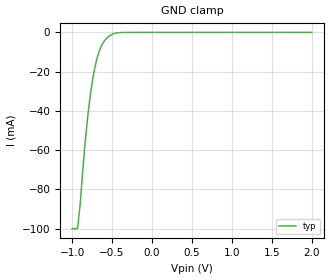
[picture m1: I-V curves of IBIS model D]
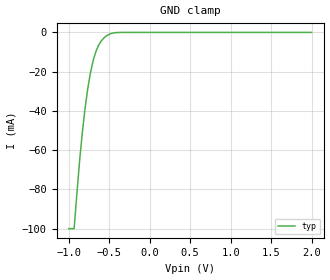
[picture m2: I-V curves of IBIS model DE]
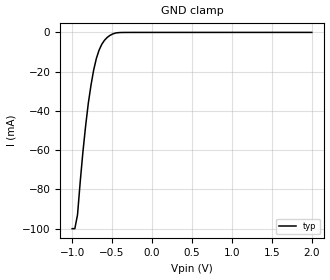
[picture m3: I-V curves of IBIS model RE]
| Texas Instruments Incorporated
| Dominant Mode Multipoint Transceiver
| Marketing part#   Voltage Range   Package-type   #pins/pkg drawing
| DS36277   4.75V - 5.25V   SOIC   8-pin D
[IBIS Ver]   4.1
[File name]   ds36277.ibs
[File Rev]   1.0
[Date]   10/01/2014
[Source]   Model built from bench measurements at:
   Texas Instruments Incorporated.
   Analog-eLab, HPA
   12500 TI Blvd
   Dallas, TX -75243
   For Support e-mail: elab_ibis@list.ti.com
[Notes]   Revision History
   Rev 1.0: 10/01/2014
   - ccomp values are based on measurement to GND.
   - R 3-state output Pullup is non-monotonic and as measured.
[Disclaimer]  This model is designed as an aid for customers of Texas Instruments
 TI and its licensors and suppliers make no warranties, either expressed
 or implied, with respect to this  model, including the warranties of
 merchantability or fitness for a particular purpose.
 The model is provided solely on an "as is" basis. The entire risk as to
 its quality and performance is with the customer.
[Copyright] (C)Copyright 2014 Texas Instruments Incorporated.
   All rights reserved.
[Component]   DS36277D
[Manufacturer]  Texas Instruments Incorporated
[Package]   |8-pin SOIC D package
|   typ   min   max
R_pkg   0   0   0
L_pkg   0   0   0
C_pkg   0   0   0
[Pin]   signal_name   model_name   R_pin   L_pin   C_pin
1   R   R
2   RE   RE
3   DE   DE
4   D   D
5   GND   GND
6   A   DO
7   B   DO
8   VCC1   POWER
[Diff pin]  inv_pin  vdiff  tdelay_typ  tdelay_min  tdelay_max
 6   7   0.0   0.0s   0.0s   0.0s
| Models and submodels in the file (5): D (Input), DE (Input), RE (Input), R (3-state), DO (I/O)
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|   Model D
[Model]   D
Model_type   Input
Vinl = .8
Vinh = 2
|   typ   min   max
|   (nom PVT)   (fast PVT)   (slow PVT)
C_comp   11.252pF   NA   NA
[Voltage Range]   5   NA   NA
[Temperature Range]   27   NA   NA
[Power Clamp Reference]   5   NA   NA
[GND Clamp Reference]   0   0   0
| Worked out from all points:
|   GND clamp passes 1 mA (typ) near -0.50 V on its own axis
[GND Clamp]
|   Voltage   I(typ)   I(min)  I(max)
-1V       -100mA     NA         NA
-932.6mV  -100mA     NA         NA
-898.9mV  -87.56mA   NA         NA
-865.2mV  -69.25mA   NA         NA
-831.5mV  -53.38mA   NA         NA
-797.8mV  -40.13mA   NA         NA
-764mV    -29.44mA   NA         NA
-730.3mV  -20.87mA   NA         NA
-662.9mV  -9.703mA   NA         NA
-561.8mV  -2.723mA   NA         NA
-359.6mV  -36.74uA   NA         NA
2V        0A         NA         NA
|   Model DE
[Model]   DE
Model_type   Input
Vinl = .8
Vinh = 2
|   typ   min   max
|   (nom PVT)   (fast PVT)   (slow PVT)
C_comp   11.252pF   NA   NA
[Voltage Range]   5   NA   NA
[Temperature Range]   27   NA   NA
[Power Clamp Reference]   5   NA   NA
[GND Clamp Reference]   0   0   0
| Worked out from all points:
|   GND clamp passes 1 mA (typ) near -0.50 V on its own axis
[GND Clamp]
|   Voltage   I(typ)   I(min)  I(max)
-1V       -100mA     NA         NA
-932.6mV  -100mA     NA         NA
-865.2mV  -65.53mA   NA         NA
-831.5mV  -51.06mA   NA         NA
-797.8mV  -38.77mA   NA         NA
-764mV    -28.58mA   NA         NA
-730.3mV  -20.45mA   NA         NA
-662.9mV  -9.664mA   NA         NA
-629.2mV  -6.458mA   NA         NA
-561.8mV  -2.706mA   NA         NA
-393.3mV  -58.84uA   NA         NA
2V        0A         NA         NA
|   Model RE
[Model]   RE
Model_type   Input
Vinl = .8
Vinh = 2
|   typ   min   max
|   (nom PVT)   (fast PVT)   (slow PVT)
C_comp   12.618pF   NA   NA
[Voltage Range]   5   NA   NA
[Temperature Range]   27   NA   NA
[Power Clamp Reference]   5   NA   NA
[GND Clamp Reference]   0   0   0
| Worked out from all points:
|   GND clamp passes 1 mA (typ) near -0.50 V on its own axis
[GND Clamp]
|   Voltage   I(typ)   I(min)  I(max)
-1V       -100mA     NA         NA
-966.3mV  -100mA     NA         NA
-932.6mV  -92.95mA   NA         NA
-865.2mV  -60.96mA   NA         NA
-831.5mV  -47.78mA   NA         NA
-797.8mV  -36.17mA   NA         NA
-730.3mV  -19.17mA   NA         NA
-696.6mV  -13.28mA   NA         NA
-662.9mV  -9.055mA   NA         NA
-561.8mV  -2.599mA   NA         NA
-393.3mV  -62.28uA   NA         NA
2V        0A         NA         NA
